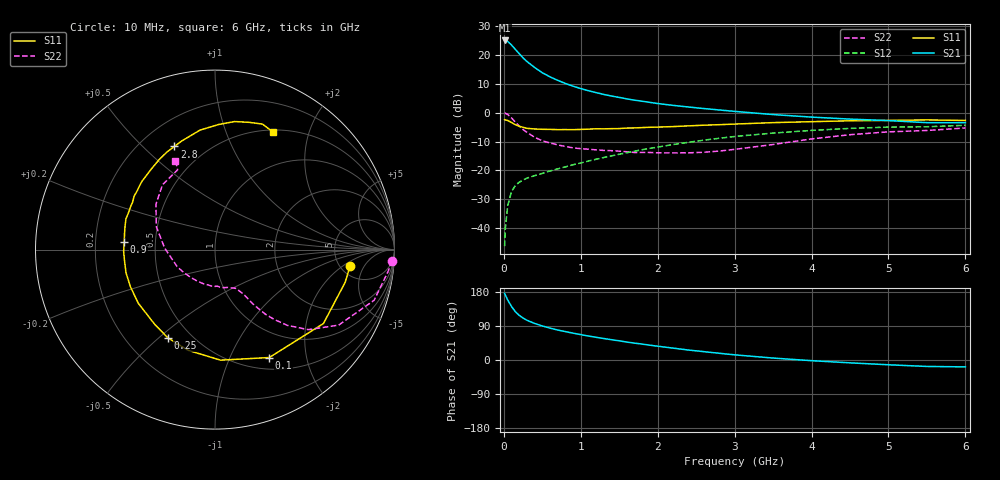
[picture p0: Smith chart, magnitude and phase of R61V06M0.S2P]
! SIEMENS Small Signal Semiconductors
! BFR193
! Si NPN RF Bipolar Junction Transistor in SOT23
! VCE = 1 V  IC = 6 mA
! Common Emitter S-Parameters:  May  1996
# GHz  S  MA  R  50
!  f  S11  S21  S12  S22
! GHz  MAG  ANG  MAG  ANG  MAG  ANG  MAG  ANG
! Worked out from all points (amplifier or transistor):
!   36 points, 10 MHz to 6 GHz, reference 50 ohm
!   highest |S21| = 25.0 dB at 10 MHz (marker M1)
!   |S21| within 3 dB of that: start of sweep to 146.9 MHz
!   unconditionally stable (mu >= 1): 822.2 MHz to 2.186 GHz
!   at 250 MHz: K = 0.49, MSG = 21.1 dB, |S12| = -23.3 dB
!   at 1.4 GHz: K = 1.07, MAG = 8.7 dB, |S12| = -15.0 dB
!   at 6 GHz: K = 0.98, MSG = 0.4 dB, |S12| = -4.4 dB
!   S11 on the Smith chart (normalised r, x): 10 MHz: 6.06, -2.66; 100 MHz: 0.64, -1.42; 250 MHz: 0.38, -0.53; 900 MHz: 0.33, +0.04; 2.8 GHz: 0.34, +0.63; 6 GHz: 0.52, +1.47
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0.01  0.7577 -7.1  17.69 175.9  0.0049 84.9  0.987 -3.6
0.02  0.7478 -14.1  17.68 171.1  0.01 83.2  0.9726 -7.1
0.05  0.7312 -34.3  17.1 158.6  0.0246 74.3  0.9301 -17.7
0.1  0.6731 -63.3  14.72 141.2  0.0432 62.0  0.8073 -31.4
0.15  0.6168 -87.1  12.39 127.3  0.055 53.9  0.6854 -40.6
0.2  0.5808 -105.0  10.44 117.8  0.0625 49.7  0.5842 -46.3
0.25  0.5571 -118.2  8.825 110.6  0.0684 47.4  0.5102 -49.7
0.3  0.5347 -129.0  7.659 104.9  0.0736 46.7  0.455 -52.1
0.4  0.5216 -145.1  6.032 96.5  0.0812 46.5  0.3744 -54.9
0.5  0.5146 -156.3  4.895 89.8  0.0888 47.9  0.3256 -56.3
0.6  0.5124 -165.4  4.153 84.2  0.0979 49.2  0.298 -57.3
0.7  0.508 -172.8  3.617 79.1  0.1064 50.9  0.2766 -58.7
0.9  0.5072 175.4  2.864 70.8  0.1255 53.5  0.2451 -62.0
1.1  0.5173 165.8  2.392 63.3  0.1455 54.9  0.2326 -66.7
1.3  0.5238 157.3  2.06 56.7  0.1674 55.4  0.2217 -71.9
1.6  0.5404 146.4  1.726 47.3  0.2023 55.0  0.2103 -82.7
2.2  0.573 128.0  1.333 31.4  0.2803 50.8  0.2009 -109.6
2.8  0.618 111.5  1.11 17.8  0.3597 43.5  0.2164 -144.2
3.5  0.6711 97.1  0.925 5.1  0.4426 32.4  0.2808 178.2
4.5  0.7218 81.3  0.772 -7.5  0.5334 16.7  0.4147 142.5
5.5  0.7477 69.3  0.67 -17.0  0.5693 1.3  0.4907 115.1
6  0.7312 64.0  0.669 -18.2  0.6036 -3.3  0.5419 114.0
